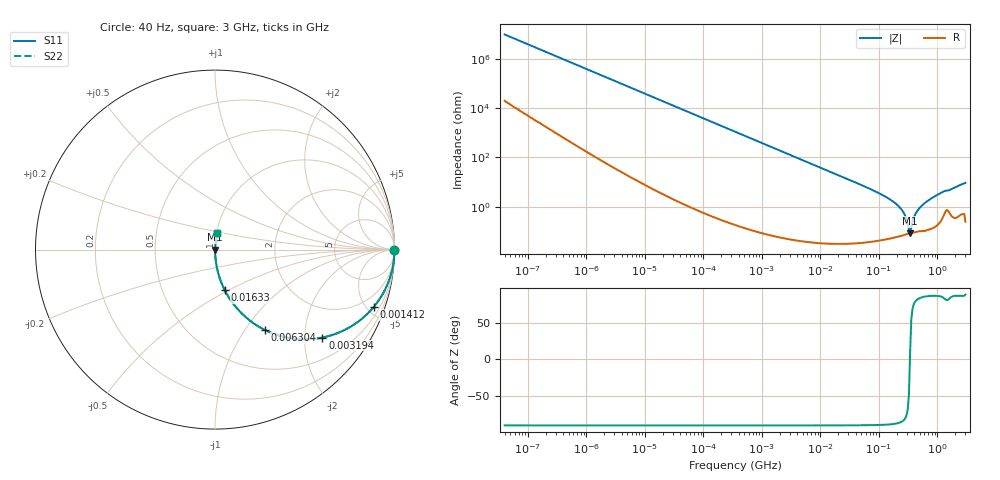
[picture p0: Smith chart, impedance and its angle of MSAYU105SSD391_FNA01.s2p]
! MSAYU105SSD391_FNA01  S-PARAMETER MODEL  ( General Type )
! Model Generated by TAIYO YUDEN Corporation (http://www.ty-top.com)
! Version 2.0
! TAIYO YUDEN Control No. 051115
! Copyright(c) 2005 TAIYO YUDEN CO.,LTD. All Rights Reserved.
! Product Description (link to TY-COMPAS)
! https://ds.yuden.co.jp/TYCOMPAS/or/detail?pn=MSAYU105SSD391KFNA01&u=M
! Products Name : Multilayer Ceramic Capacitors
! Characteristics :
!  Capacitance : 390 pF , Rated Voltage : 50V
!  Case Size : 1.0 x 0.5 / 0.039 x 0.02 [mm/inch] , Thickness : 0.5 / 0.02 [mm/inch]
!  (Conditions: Temperature = 25 degC , DC Bias Current/Voltage = 0A / 0V)
! External Node Assignments :
!  1  o---| |---o  2
! GND o---------o GND
! Frequency Range : 40Hz  -  3GHz  [ 401 STEP ]
# MHz S RI R 50
! Freq[MHz].  S11 Real  S11 Imag  S21 Real  S21 Imag  S12 Real  S12 Imag  S22 Real  S22 Imag
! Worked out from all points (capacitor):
!   401 points, 40 Hz to 3 GHz, reference 50 ohm
!   read as one part in series: C = 408 pF near 44 Hz
!   lowest |Z| = 85.3 mohm at 340.5 MHz (marker M1)
!   series resonance near 338.7 MHz, so ESL is about 540 pH
!   S11 on the Smith chart (normalised r, x): 40 Hz: open; 1.412 MHz: 1.00, -5.52; 3.194 MHz: 1.00, -2.44; 6.304 MHz: 1.00, -1.24; 16.33 MHz: 1.00, -0.48; 3 GHz: 1.00, +0.19
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4e-05  1 -1.03e-05  2.1e-08 1.03e-05  2.1e-08 1.03e-05  1 -1.03e-05
0.000369  1 -9.46e-05  7.3e-08 9.46e-05  7.3e-08 9.46e-05  1 -9.46e-05
0.000834  1 -0.000214  1.47e-07 0.000214  1.47e-07 0.000214  1 -0.000214
0.017386  1 -0.00446  2.06e-05 0.00446  2.06e-05 0.00446  1 -0.00446
0.362475  0.9914 -0.0921  0.00858 0.0921  0.00858 0.0921  0.9914 -0.0921
1.412238  0.884 -0.3201  0.116 0.3201  0.116 0.3201  0.884 -0.3201
3.193638  0.5986 -0.49  0.4014 0.49  0.4014 0.49  0.5986 -0.49
6.303771  0.2768 -0.4471  0.7232 0.4471  0.7232 0.4471  0.2768 -0.4471
7.222098  0.2258 -0.4178  0.7742 0.4178  0.7742 0.4178  0.2258 -0.4178
16.33207  0.054 -0.2253  0.946 0.2253  0.946 0.2253  0.054 -0.2253
69.67004  0.00323 -0.0534  0.9968 0.0534  0.9968 0.0534  0.00323 -0.0534
150.5692  0.00093 -0.0206  0.9991 0.0206  0.9991 0.0206  0.00093 -0.0206
247.9136  0.000724 -0.00722  0.9993 0.00722  0.9993 0.00722  0.000724 -0.00722
284.0294  0.000762 -0.00402  0.9992 0.00402  0.9992 0.00402  0.000762 -0.00402
310.9844  0.000802 -0.00194  0.9992 0.00194  0.9992 0.00194  0.000802 -0.00194
340.4975  0.000844 0.000119  0.9992 -0.000119  0.9992 -0.000119  0.000844 0.000119
356.2883  0.00087 0.00117  0.9991 -0.00117  0.9991 -0.00117  0.00087 0.00117
408.192  0.000936 0.00429  0.9991 -0.00429  0.9991 -0.00429  0.000936 0.00429
446.9303  0.00101 0.00642  0.999 -0.00642  0.999 -0.00642  0.00101 0.00642
613.8375  0.00126 0.0144  0.9987 -0.0144  0.9987 -0.0144  0.00126 0.0144
1211.625  0.00488 0.0387  0.9951 -0.0387  0.9951 -0.0387  0.00488 0.0387
3000  0.011 0.0919  0.989 -0.0919  0.989 -0.0919  0.011 0.0919
